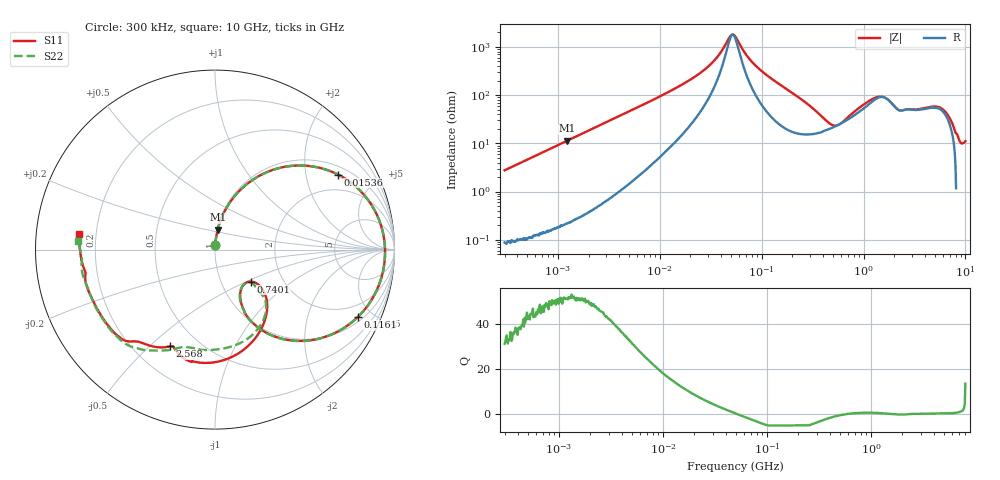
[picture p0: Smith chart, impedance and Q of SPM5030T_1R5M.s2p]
! S-Parameter Data Generated by TDK Corporation
! Copyright(C) 2019 TDK Corporation.
! All Rights Reserved.
! TDK P/N: SPM5030T-1R5M (Inductor)
! Property: L=1.5uH at 100kHz
! Size(LxWxT): 5.2x5x3mm
! Model Type: s2p (Touchstone File Format Version 1.0)
! Frequency: DC=Yes Start=0.3MHz Stop=10000MHz 802points Log-sweep
! Model Generated on Sep. 23, 2019
! Port Assignments:
!  1 ---@@@--- 2
! Applicable Conditions:
!  Temperature = 25 degC
!  DC Bias Current = 0 A
!  Small Signal Operation
! Terms and conditions regarding TDK Simulation Models
! (1)This simulation model is being provided solely for informational purposes. Please refer to the specifications of the products in terms of detailed characteristics of such products.
! (2)In no event shall TDK Corporation of any of its subsidiaries be liable for any loss or damage arising, directly or indirectly,
!  From any information contained in this simulation model, including, but not limited to loss or damages arising from any inaccuracies, omissions or errors in connection with such information.
! (3)Any and all copyrights on this simulation model are owned by TDK Corporation.
!  Duplication or redistribution of this simulation model without prior written permission from TDK Corporation is prohibited.
! (4)This simulation model is subject to any modification or change without any prior notice.
! (5)Neither TDK Corporation nor any of its subsidiaries shall make any warranty, express or implied,
!  Including but not limited to the correctness, implied warranties of merchantability and fitness for a particular purpose with respect to this simulation models.
! (6)The use of this simulation model shall be deemed to have consented to the terms and conditions hereof.
# Hz S MA R 50
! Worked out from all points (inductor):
!   801 points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, 300 kHz to 10 GHz, reference 50 ohm
!   read as one part in series: L = 1.46 uH near 318.3 kHz
!   highest Q = 51.8 at 1.238 MHz (marker M1), where L = 1.46 uH
!   self-resonance near 52.07 MHz
!   S11 on the Smith chart (normalised r, x): 300 kHz: 1.00, +0.05; 15.36 MHz: 1.30, +3.06; 116.1 MHz: 1.24, -4.11; 740.1 MHz: 1.38, -0.53; 2.568 GHz: 0.35, -0.58; 10 GHz: 0.13, +0.05
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300000  0.02727 86.5  0.9987 -1.6  0.9988 -1.6  0.02722 86.5
1237570  0.112 82.4  0.9915 -6.5  0.9916 -6.5  0.112 82.4
1713600  0.1539 79.9  0.9851 -8.9  0.9851 -8.9  0.1539 80.0
4425256  0.3708 66.4  0.9179 -21.9  0.9179 -21.9  0.3708 66.4
9671944  0.6529 45.8  0.7234 -41.1  0.7233 -41.1  0.6529 45.8
1.535588e7  0.8029 31.4  0.5324 -53.8  0.5324 -53.8  0.8029 31.4
2.987769e7  0.9229 12.1  0.2362 -65.7  0.2362 -65.7  0.923 12.0
4.929468e7  0.9476 -0.9  0.05662 -24.0  0.05663 -24.0  0.9477 -0.9
5.477226e7  0.9473 -3.6  0.05632 17.9  0.05632 17.9  0.9475 -3.6
7.683413e7  0.9332 -12.6  0.1702 59.0  0.1702 59.0  0.9334 -12.6
1.161426e8  0.8798 -25.3  0.3513 55.2  0.3513 55.2  0.8799 -25.3
1.945824e8  0.7278 -44.0  0.5891 37.7  0.5891 37.7  0.7279 -44.1
3.126428e8  0.5059 -60.5  0.7519 15.9  0.7519 15.9  0.5058 -60.7
4.866838e8  0.3021 -62.3  0.7938 -6.4  0.7939 -6.4  0.3018 -62.8
7.400828e8  0.2674 -41.7  0.7248 -28.4  0.7249 -28.4  0.2649 -43.6
1.24442e9  0.4777 -54.2  0.5016 -50.2  0.5017 -50.2  0.4567 -52.2
1.767019e9  0.6238 -88.2  0.4022 -49.3  0.4021 -49.3  0.5557 -88.1
2.568366e9  0.5943 -114.9  0.414 -69.6  0.4139 -69.6  0.5942 -111.7
4.690952e9  0.7145 -134.9  0.2456 -103.9  0.2455 -103.9  0.7139 -130.8
6.010849e9  0.7286 -141.6  0.2009 -114.7  0.2009 -114.6  0.7337 -143.1
8.770142e9  0.7463 -175.5  0.1407 -146.7  0.1408 -146.7  0.754 178.9
1e10  0.7642 173.6  0.1131 -154.4  0.1132 -154.4  0.7625 176.4
